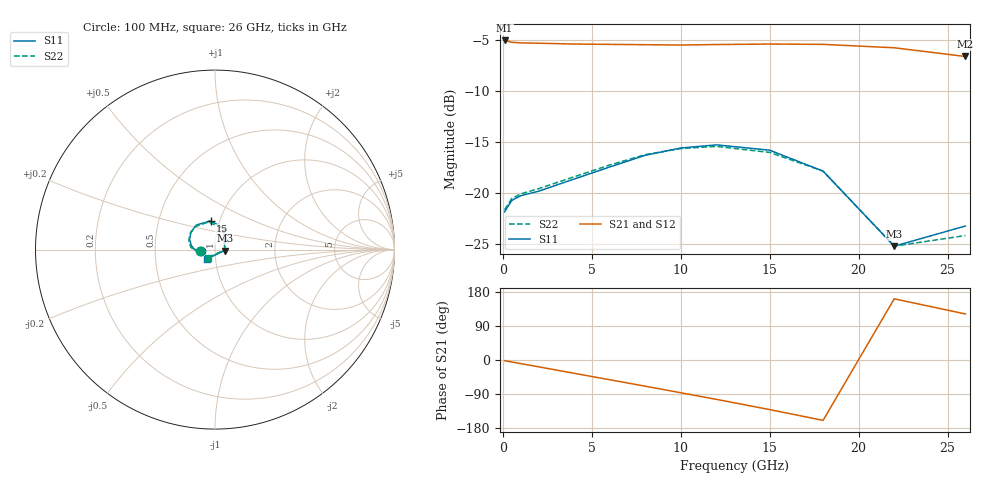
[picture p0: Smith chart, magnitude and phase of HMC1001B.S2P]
! HMMC-1001
! Typical s-parameters at 5dB attenuation setting, TA = 25 C
# ghz s ma r 50
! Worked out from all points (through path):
!   13 points, 100 MHz to 26 GHz, reference 50 ohm
!   highest |S21| = -5.08 dB at 100 MHz (marker M1); lowest = -6.7 dB at 26 GHz (marker M2)
!   lowest |S11| = -25.2 dB at 22 GHz (marker M3), VSWR 1.12, Z = 55.8 - j0.579 ohm
!   |S11| at or under -10 dB: start of sweep to end of sweep
!   |S22| runs from -25.2 to -15.4 dB; largest |S21 - S12| = 0.0056
!   S11 on the Smith chart (normalised r, x): 100 MHz: 0.85, -0.01; 15 GHz: 0.91, +0.30; 26 GHz: 0.91, -0.09
0.1  0.081 -173.8  0.557 -1.8  0.557 -1.8  0.083 -173.5
0.5  0.092 -175.0  0.546 -5.3  0.545 -5.1  0.094 -175.2
1  0.097 -176.9  0.542 -9.4  0.541 -9.3  0.099 -175.9
2  0.102 -178.0  0.54 -17.9  0.539 -17.8  0.105 -176.3
4  0.117 178.4  0.535 -35.0  0.535 -34.9  0.12 -179.2
6  0.134 170.1  0.533 -52.0  0.532 -52.0  0.137 173.2
8  0.153 158.0  0.531 -69.1  0.53 -69.2  0.154 161.3
10  0.166 143.5  0.529 -86.4  0.53 -86.5  0.165 147.1
12  0.172 126.9  0.532 -103.8  0.531 -103.8  0.169 130.6
15  0.162 98.7  0.535 -130.9  0.534 -130.8  0.158 103.4
18  0.128 66.6  0.533 -159.3  0.532 -159.1  0.128 69.8
22  0.055 -5.4  0.513 161.4  0.514 161.3  0.055 -0.7
26  0.069 -131.1  0.465 121.5  0.47 121.2  0.062 -132.2
